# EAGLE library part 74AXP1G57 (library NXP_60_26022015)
Low-power configurable gate with voltage-level translator The 74AXP1G57 is a configurable multiple function gate with Schmitt-trigger inputs. The device can be configured as any of the following logic functions AND, OR, NAND, NOR, XNOR, inverter and buffer. All inputs can be connected directly to VCC or GND. This device ensures very low static and dynamic power consumption across the entire VCC range from 0.7 V to 2.75 V. This device is fully specified for partial power down applications using IOFF. The IOFF circuitry disables the output, preventing the potentially damaging backflow current through the device when it is powered down. AAL Eindhoven MK
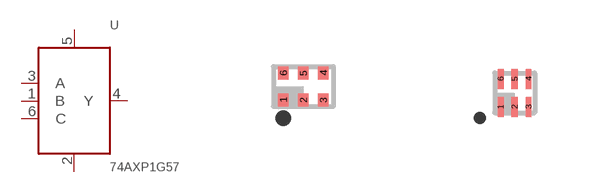
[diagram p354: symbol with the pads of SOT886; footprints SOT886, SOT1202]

Designator prefix U

## 74AXP1G57GM  [SOT886]
1  B  in
2  GND  pwr
3  A  in
4  Y  out
5  VCC  pwr
6  C  in

## 74AXP1G57GS  [SOT1202]
Pads as for SOT886

## 74AXP1G57GN  [SOT1115]
Pads as for SOT886

## Footprint SOT886 (pad centres in mm)
SOT886 XSON6: plastic extremely thin small outline package; no leads; 6 terminals; body 1 x 1.45 x 0.5 mm JEDEC: MO-252 IEC: ---
smd 0.27 x 0.325: 1 -0.5,-0.338; 2 0,-0.338; 3 0.5,-0.338; 4 0.5,0.338; 5 0,0.338; 6 -0.5,0.338

## Footprint SOT1202 (pad centres in mm)
SOT1202 XSON6: extremely thin small outline package; no leads; 6 terminals; body 1.0 x 1.0 x 0.35 mm JEDEC: --- IEC: ---
smd 0.15 x 0.5: 1 -0.35,-0.35; 2 0,-0.35; 3 0.35,-0.35; 4 0.35,0.35; 5 0,0.35; 6 -0.35,0.35

## Footprint SOT1115 (pad centres in mm)
!!!!!!Experimental, not tested!!!!!!!!!!!! MK SOT1115 XSON6: extremely thin small outline package; no leads; 6 terminals; body 0.9 x 1.0 x 0.35 mm JEDEC: -- IEC: -- JEITA: --
smd 0.22 x 0.325: 1 -0.3,-0.312; 2 0,-0.312; 3 0.3,-0.312; 4 0.3,0.312; 5 0,0.312; 6 -0.3,0.312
